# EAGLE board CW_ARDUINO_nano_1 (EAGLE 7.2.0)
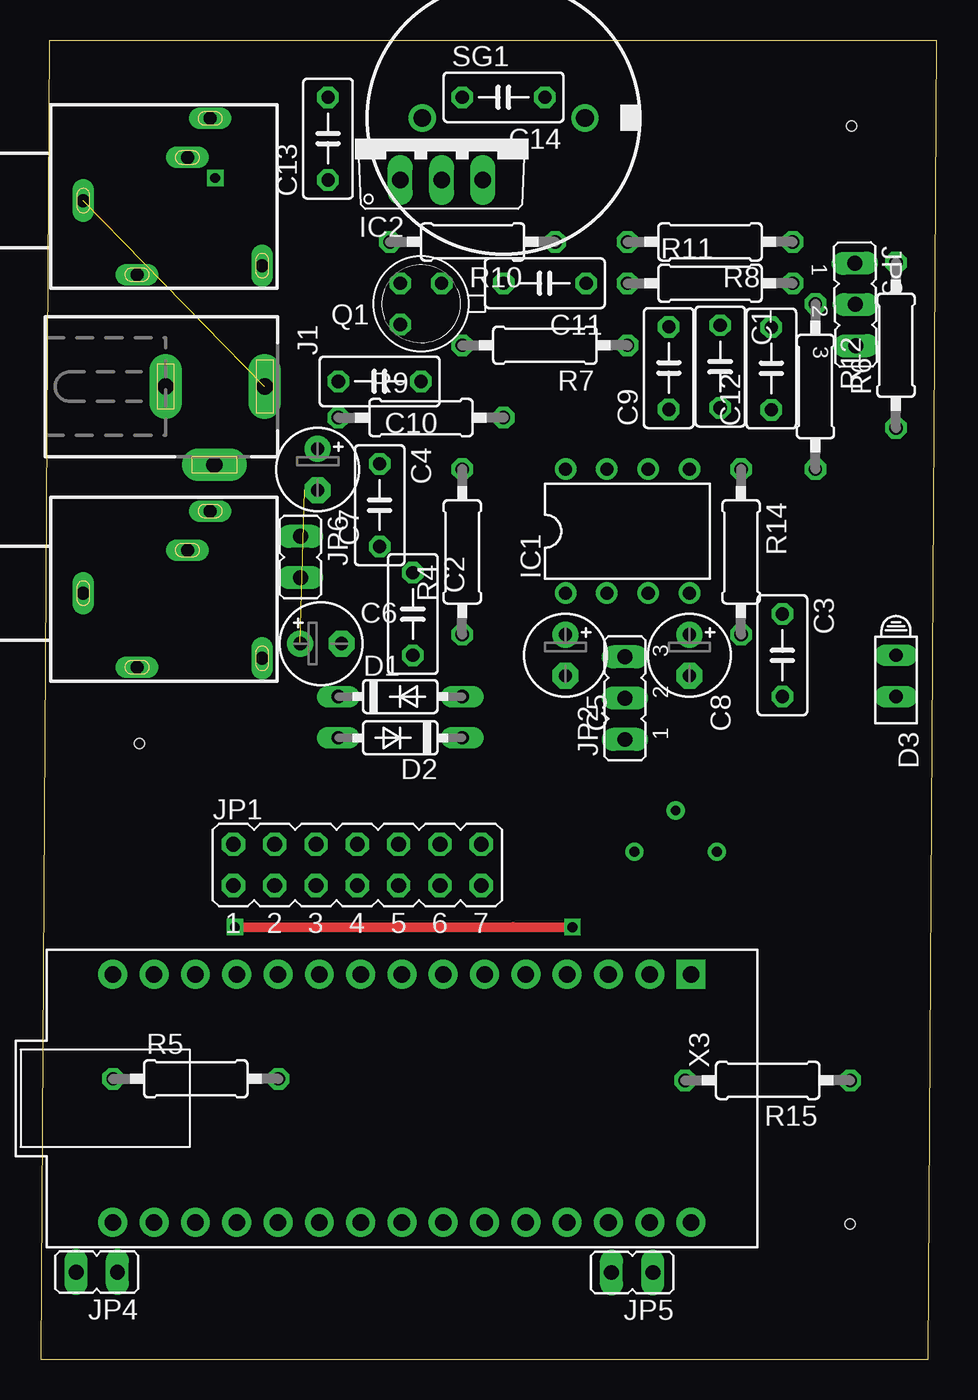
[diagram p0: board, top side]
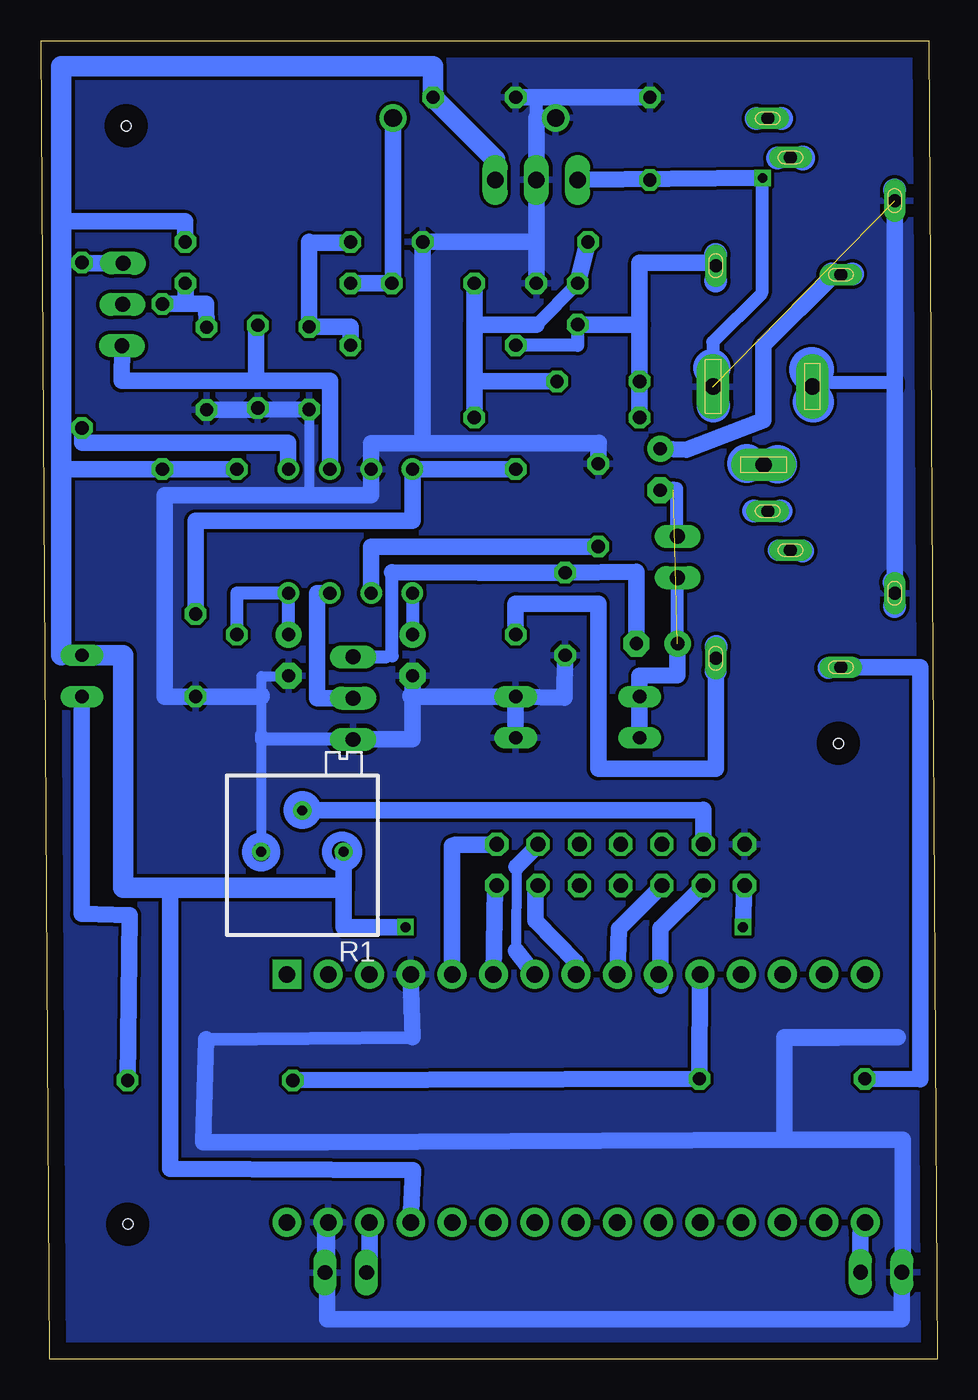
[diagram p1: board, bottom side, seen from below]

Size 55.12 x 81.05 mm. Coordinates in mm from the lower left corner, seen from the top.
Outline: 0,0 54.59,0 55.12,81.05 0.53,81.05 0,0
Copper layers (1*16): Top 0.035mm / dielectric 1.5mm / Bottom 0.035mm
Design rules "default": minimum track width 10mil, minimum drill 24mil, track to track 8mil, track to pad 8mil, pad to pad 8mil, via to via 8mil, smd to smd 8mil, copper to edge 40mil, drill to drill 8mil, minimum pad ring 10mil, minimum via ring 8mil, stop-mask expansion 4mil, vias tented up to drill 0mil, thermal gap 10mil
Holes 0.6 mm at 49.88,75.81 49.77,8.31 6.07,37.86

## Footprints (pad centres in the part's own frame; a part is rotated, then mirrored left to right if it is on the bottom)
C050-030X075 = drill 0.813 octagon: 1 -2.54,0; 2 2.54,0
E2,5-5 = drill 0.813 pad 1.6: + -1.27,0 | drill 0.813 pad 1.6 octagon: - 1.27,0
DO35-7 = drill 0.813 long: A 3.81,0; C -3.81,0
HLMP6 = drill 0.813 long: A -1.27,0; K 1.27,0
DIL08 = drill 0.813 pad 1.27: 1 -3.81,-3.81; 2 -1.27,-3.81; 3 1.27,-3.81; 4 3.81,-3.81; 5 3.81,3.81; 6 1.27,3.81; 7 -1.27,3.81; 8 -3.81,3.81
TO220V = drill 1.016 long: 1 -2.54,-2.54; 2 0,-2.54; 3 2.54,-2.54
DCJ0202 = drill 1 pad 2 long: 1 0,3.1; 2 4.8,0; 3 0,-3
JP7Q = drill 0.914 octagon: 1 -7.62,-1.27; 2 -7.62,1.27; 3 -5.08,-1.27; 4 -5.08,1.27; 5 -2.54,-1.27; 6 -2.54,1.27; 7 0,-1.27; 8 0,1.27; 9 2.54,-1.27; 10 2.54,1.27; 11 5.08,-1.27; 12 5.08,1.27; 13 7.62,-1.27; 14 7.62,1.27
JP2 = drill 0.914 long: 1 -2.54,0; 2 0,0; 3 2.54,0
JP1 = drill 0.914 long: 1 0,-1.27; 2 0,1.27
TO18 = drill 0.813 octagon: 1 -1.27,-1.27; 2 1.27,-1.27; 3 1.27,1.27
RTRIM3296P = drill 0.61: 1 0,-2.54; 2 2.54,0; 3 0,2.54
0207/10 = drill 0.813 octagon: 1 -5.08,0; 2 5.08,0
EFBAA40D101 = drill 1.1 pad 1.676: 1 -5,0; 2 5,0
1503_09 = drill 0.8 pad 1.2 long: 1 0,-2.1; 2 -4.55,-5.4; 3 5.05,-9.9; 4 -4,-13.1; 5 2.65,-8.5
ARDUINO_NANO_C = drill 1.016 pad 1.778 square: 1 -7.62,16.51 | drill 1.016 pad 1.778: 2 -7.62,13.97; 3 -7.62,11.43; 4 -7.62,8.89; 5 -7.62,6.35; 6 -7.62,3.81; 7 -7.62,1.27; 8 -7.62,-1.27; 9 -7.62,-3.81; 10 -7.62,-6.35; 11 -7.62,-8.89; 12 -7.62,-11.43; 13 -7.62,-13.97; 14 -7.62,-16.51; 15 -7.62,-19.05; 16 7.62,-19.05; 17 7.62,-16.51; 18 7.62,-13.97; 19 7.62,-11.43; 20 7.62,-8.89; 21 7.62,-6.35; 22 7.62,-3.81; 23 7.62,-1.27; 24 7.62,1.27; 25 7.62,3.81; 26 7.62,6.35; 27 7.62,8.89; 28 7.62,11.43; 29 7.62,13.97; 30 7.62,16.51

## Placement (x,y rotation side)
C1  M1  [C050-030X075]  41.79,61.02 270 top
C2  10n  [C050-030X075]  22.89,45.8 270 top
C3  10n  [C050-030X075]  45.61,43.28 270 top
C4  M2  [C050-030X075]  20.85,52.5 270 top
C5  1u  [E2,5-5]  32.27,43.28 270 top
C6  1u  [E2,5-5]  17.24,43.99 0 top
C7  1u  [E2,5-5]  17.04,54.69 270 top
C8  10u  [E2,5-5]  39.9,43.28 270 top
C9  M1  [C050-030X075]  38.62,60.92 90 top
C10  100  [C050-030X075]  20.85,60.1 180 top
C11  10n  [C050-030X075]  31.01,66.14 180 top
C12  33n  [C050-030X075]  44.93,60.9 90 top
C13  M1  [C050-030X075]  17.67,75.03 90 top
C14  M1  [C050-030X075]  28.46,77.56 180 top
D1  1N4148  [DO35-7]  22.12,40.73 0 top
D2  1N4148  [DO35-7]  22.12,38.2 180 top
D3  HLMP6  [HLMP6]  52.59,42.01 270 top
IC1  LM567N  [DIL08]  36.09,50.9 0 top
IC2  7805TV  [TO220V]  24.66,75.03 0 top
J1  DCJ0202  [DCJ0202]  10.69,59.79 270 top
JP1  [JP7Q]  19.47,30.39 0 top
JP2  [JP2]  35.93,40.64 90 top
JP3  [JP2]  50.1,64.84 270.8 top
JP4  [JP1]  3.45,5.36 90 top
JP5  [JP1]  36.38,5.33 90 top
JP6  [JP1]  15.97,49.31 180 top
Q1  2N2222  [TO18]  23.39,64.87 180 top
R1  [RTRIM3296P]  39.05,31.19 90 bottom
R4  100  [0207/10]  25.93,49.62 90 top
R5  100  [0207/10]  9.54,17.24 0 top
R6  5k1  [0207/10]  52.59,62.33 90 top
R7  10k  [0207/10]  31.01,62.33 180 top
R8  1k  [0207/10]  41.16,68.67 180 top
R9  360k  [0207/10]  23.39,57.88 0 top
R10  110k  [0207/10]  26.56,68.67 180 top
R11  15k  [0207/10]  41.16,66.14 0 top
R12  1k  [0207/10]  47.65,59.79 270 top
R14  100  [0207/10]  43.07,49.62 270 top
R15  470  [0207/10]  44.7,17.14 180 top
SG1  mic  [EFBAA40D101]  28.46,76.3 0 top
X1  1503_09  [1503_09]  0.53,71.22 90 top
X2  1503_09  [1503_09]  0.53,47.09 90 top
X3  [ARDUINO_NANO_C]  23.49,16.04 270 top

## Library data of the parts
C1-C14 R1 R4-R12 R14 R15 = rcl
D1 D2 = diode
D3 = display-hp; MF: AGILENT TECHNOLOGIES; MPN: HLMP-6500; OC_FARNELL: 1652490; OC_NEWARK: 40K0088
IC1 IC2 = linear
J1 = con-jack; OC_FARNELL: unknown; OC_NEWARK: unknown
JP1-JP6 = jumper
Q1 = transistor-npn
SG1 = buzzer; OC_FARNELL: unknown; OC_NEWARK: unknown
X1 X2 = con-lumberg; OC_FARNELL: 1243244; OC_NEWARK: unknown
X3 = Arduino_FB

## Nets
+5V: C14.1 D3.A IC2.3 JP1.1 R1.1 R8.1 R12.2 R14.1 X3.27
N1: C1.2 C2.2 C3.2 C4.1 C5.- C8.- C9.1 C12.1 C13.2 C14.2 D1.A D2.C IC1.7 IC2.2 J1.1 JP1.2 JP2.1 JP4.2 JP5.1 Q1.1 R1.3 R10.1 SG1.1 X1.1 X2.1 X3.4 X3.29
N$1: C13.1 IC2.1
N$2: JP1.4 R1.2
N$3: JP4.1 X3.16
N$4: JP1.3 X3.10
N$5: IC1.3 JP2.2
N$6: JP1.5 X3.9
N$7: C8.+ IC1.4 R14.2
N$8: R4.1 X2.4
N$9: D3.K R15.1
N$10: JP3.1 R6.2
N$11: IC1.5 R6.1
N$12: C1.1 IC1.6 JP3.3
N$13: C3.1 IC1.8 R4.2
N$14: R5.1 X2.2
N$15: C4.2 IC1.2
N$16: JP1.14 X3.5
N$17: C5.+ IC1.1
N$18: JP1.12 X3.7
N$19: R5.2 R15.2 X3.11
N$20: C2.1 C6.- JP2.3
N$21: JP1.13 X3.6
N$22: JP1.11 X3.8
N$23: C6.+ C7.- D1.C D2.A
N$24: C10.2 Q1.3 R7.2 R9.1 X1.4
N$25: C7.+ X1.2
N$26: C9.2 R7.1 R8.2
N$27: C10.1 C11.2 Q1.2 R9.2 R10.2
N$28: C12.2 R11.2 R12.1
N$29: C11.1 R11.1 SG1.2
N$30: JP5.2 X3.28
S$5: J1.3

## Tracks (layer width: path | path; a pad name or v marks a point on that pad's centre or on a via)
+5V  (via drill 0.6)
  Top 0.61: v11.95,26.56 29.05,26.58 v32.7,26.56
  Bottom 0.406: 53.87,54.71 53.87,54.73
  Bottom 0.61: 42.28,28.99 47.19,29.08 | 36.51,28.93 37.02,28.99
  Bottom 0.813: 53.87,43.28 D3.A
  Bottom 1.016: R14.1 R12.2 53.87,54.71 | X3.27 32.25,11.62 47.19,11.72 47.19,29.08 42.38,28.98 | R8.1 46.25,69.95 53.87,69.95 | R1.1 36.51,28.93 36.51,26.56 v32.7,26.56 | JP1.1 11.87,29.12 11.9,29.04 11.92,26.58 v11.95,26.56
  Bottom 1.27: IC2.3 27.2,73.75 C14.1 31.01,79.47 53.87,79.47 53.87,69.95 53.87,54.73 53.87,43.28 | D3.A 50.05,43.28 50.05,28.98 42.38,28.98 | 37.02,28.99 42.28,28.99
N1  (1 unrouted)
  Bottom 0.406: X3.29 37.53,8.42
  Bottom 0.61: C9.1 38.62,53.12 | R1.3 41.55,31.19 41.55,38.36 41.55,40.81 41.55,41.98 39.9,41.98 C8.-
  Bottom 0.813: IC2.2 24.66,75.34 | 24.66,76.3 24.66,77.56 | 44.95,19.68 32.27,19.78 | JP2.1 41.55,38.09 41.55,38.36
  Bottom 1.016: Q1.1 24.66,68.67 | 24.66,68.67 IC2.2 24.66,76.3 SG1.1 | 24.66,68.67 R10.1 31.64,56.29 | X1.1 X2.1 | 31.64,56.29 34.82,56.29 IC1.7 34.82,53.12 38.62,53.12 47.52,53.12 47.52,40.73 C3.2 41.55,40.73 41.55,40.81 | 31.64,56.29 20.85,56.29 | 20.85,56.29 20.81,56.34 | C4.1 20.85,56.29 | D2.C D1.A | C9.1 41.85,58.37 | 41.85,58.37 C12.1 | C13.2 24.66,77.56 C14.2 | 44.95,19.68 45.16,13.33 37.53,13.35 9.41,13.48 9.41,19.78 2.43,19.78 | 32.27,19.78 X3.4 | C2.2 22.93,40.66 D1.A | C1.2 41.85,58.48 41.85,58.37 | 2.62,19.81 9.4,19.73 9.4,13.49 2.12,13.49 2.12,4.61 JP4.2 2.18,2.46 37.52,2.46 37.52,8.42 X3.29 37.65,8.42 JP5.1 | D1.A 32.4,40.73 32.4,40.81 32.27,40.81 C5.- 32.27,38.09 JP2.1
  pour Bottom: 0.57,81.03 55.23,81.03 55.52,0.49 0.92,0.49 0.62,81.01
N$1  (via drill 0.6)
  Bottom 0.406: C13.1 IC2.1
  Bottom 1.016: IC2.1 v10.73,72.61
N$2
  Bottom 1.016: R1.2 14.43,33.73 14.38,33.79 14.38,31.67 JP1.4
N$3
  Bottom 1.016: X3.16 4.74,7.71 JP4.1
N$4
  Bottom 1.016: X3.10 17.03,22.95 17.03,26.48 JP1.3
N$5
  Bottom 1.016: IC1.3 38.12,47.09 38.12,40.64 JP2.2
N$6
  Bottom 1.016: X3.9 19.58,26.47 JP1.5
N$7
  Bottom 0.813: R14.2 43.07,47.09 IC1.4 C8.+
N$8
  Bottom 1.016: R4.1 25.93,46.45 20.85,46.45 20.85,36.29 13.6,36.29 13.6,43.14 X2.4
N$9
  Bottom 1.016: D3.K 52.62,40.73 52.62,27.38 49.66,27.29 R15.1
N$10
  Bottom 0.813: R6.2 52.37,67.41
  Bottom 1.016: JP3.1 52.59,67.38 R6.2
N$11
  Bottom 1.016: IC1.5 39.93,54.71 39.93,56.34 52.59,56.34 R6.1
N$12
  Bottom 1.016: IC1.6 37.35,60.14 41.88,60.14 | 41.88,60.14 50.16,60.14 JP3.3 | C1.1 41.88,63.55 41.88,60.14
N$13
  Bottom 1.016: C3.1 45.61,51.53 32.27,51.53 IC1.8 R4.2
N$14
  Bottom 1.016: X2.2 1.06,42.54 1.06,17.21 R5.1
N$15
  Bottom 1.016: C4.2 34.82,49.96 IC1.2
N$16
  Bottom 1.016: X3.5 29.84,31.57 29.65,31.63 27.11,31.63 JP1.14
N$17
  Bottom 0.813: IC1.1 C5.+
N$18
  Bottom 0.61: 25.88,30.26 25.9,25.1
  Bottom 1.016: JP1.12 24.55,31.58 25.88,30.26 | 25.9,25.1 X3.7
N$19
  Bottom 1.016: X3.11 R5.2 R15.2
N$20
  Bottom 0.254: C2.1 23.03,48.39 23.03,48.34
  Bottom 0.406: 33.93,43.18 33.93,43.23 33.52,43.23 | 28.18,48.34 28.16,48.34
  Bottom 0.813: JP2.3 33.93,43.18 | 33.52,43.23 33.52,48.36
  Bottom 1.016: C6.- 18.51,48.39 23.03,48.34 28.16,48.34 | 33.52,48.36 28.18,48.34
N$21
  Bottom 1.016: X3.6 27.2,29.01 JP1.13
N$22
  Bottom 1.016: X3.8 22.21,24.4 24.7,26.96 24.7,28.97 JP1.11
N$23  (1 unrouted)
  Bottom 1.016: C7.- 16.24,53.45 | C6.+ 15.99,42.03 18.3,42.01 D1.C D2.A
N$24
  Bottom 0.813: 13.62,67.41 X1.4 | Q1.3 22.12,62.33 R7.2
  Bottom 1.016: R9.1 C10.2 18.3,63.59 | 18.3,63.59 18.3,67.41 13.62,67.41 | Q1.3 18.3,63.59
N$25
  Bottom 1.016: X1.2 6.34,66.67 10.69,62.33 10.69,57.72 15.44,55.91 C7.+
N$26
  Bottom 0.254: 36.27,68.64 R8.2
  Bottom 1.016: 38.62,68.64 C9.2 36.09,63.46 R7.1 | 38.62,68.64 38.62,68.67 | 38.62,68.64 36.27,68.64
N$27
  Bottom 0.813: 24.66,63.59 Q1.2
  Bottom 1.016: R10.2 Q1.2 | C11.2 28.46,63.59 | 28.46,63.59 24.66,63.59 | R9.2 28.46,60.1 | 28.46,60.1 28.46,63.59 | C10.1 28.46,60.1
N$28
  Bottom 1.016: R12.1 46.23,64.87 | 46.23,64.87 44.95,64.87 C12.2 | R11.2 46.23,66.14 46.23,64.87
N$29
  Bottom 0.813: C11.1 33.47,66.14
  Bottom 1.016: R11.1 C11.1 | 33.47,66.14 SG1.2
N$30
  Bottom 1.016: JP5.2 34.91,5.33 X3.28
S$1
  Bottom 0.813: 7.67,60.06 2.6,60.06 2.6,59.76
S$2
  Bottom 0.813: 15.9,50.59 16.03,50.59 16.03,53.51
S$3
  Bottom 0.813: 15.97,44.04 15.97,48.11
S$5
  Top 0.406: 7.51,60.59 J1.3
S$6
  Bottom 0.813: 10.8,72.53 10.8,65.53 13.8,62.54 13.8,60.94 13.85,60.89 13.85,58.89 13.8,58.84
(copper drawn outside any net)
  shapes: Bottom circle x29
